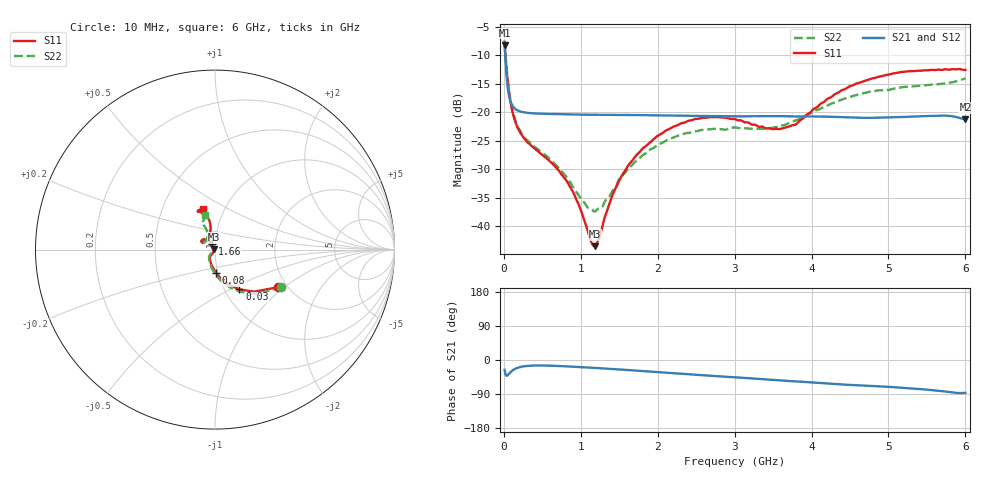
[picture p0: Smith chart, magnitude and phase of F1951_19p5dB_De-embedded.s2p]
! Integrated Device Technology
! Corporate Headquarters
! 6024 Silver Creek Valley Road
! San Jose, CA 95138  USA
! Phone:  1-408-284-8200
! Toll Free:  1-800-223-1366
! Webpage:  http://www.idt.com/
! Timing and RF Division
! 515 Groton Road, Suite 102
! Westford, MA 01886-6024
! Device:  F1951
! Description: 6-bit 0.5 dB Digital Step Attenuator
! Frequency:  100.0 -  4000.00 MHz
! Package:  4x4 mm Thin QFN Plastic Package: 24 pin
! Ports:  2 RF, 6 DC
!  Pin  1  = NC
!  Pin  2  = RF1  =  Port 1
!  Pin  3  = GND
!  Pin  4  = NC
!  Pin  5  = Serial Data Out (SDO)
!  Pin  6  = NC
!  Pin  7  = Reset Bar ( RSTb)
!  Pin  8  = Clock (CLK)
!  Pin  9  = Chip Select Bar (CSb)
!  Pin 10  = NC
!  Pin 11  = Serial Data In (SDI)
!  Pin 12  = NC
!  Pin 13  = NC
!  Pin 14  = VDD
!  Pin 15  = NC
!  Pin 16  = GND
!  Pin 17  = RF2  =  Port 2
!  Pin 18  = NC
!  Pin 19  = GND
!  Pin 20  = GND
!  Pin 21  = GND
!  Pin 22  = GND
!  Pin 23  = GND
!  Pin 24  = GND
! State:  39
! Atten State:  19.5 dB
! Voltage:  +3.30 Volts
! Current:  0.485 mA
! Data:  The device was measured on a F195X evaluation board which has
!  individual transmission lines to the RF pins.  Data was collected
!  de-embedded using a Automatic Fixture Removal [AFR] (Keysight Technologies).
!  The reference plane is the edge of the package pin.
! Misc:  Lot Code  1225BCA
!  Action Tracker AT0399
! Date Measured:  2018-09-13
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# GHz S dB R 50
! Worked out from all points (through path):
!   600 points, 10 MHz to 6 GHz, reference 50 ohm
!   highest |S21| = -8.24 dB at 10 MHz (marker M1); lowest = -21.3 dB at 6 GHz (marker M2)
!   group delay of S21, straight-line fit = 34.4 ps
!   lowest |S11| = -43.5 dB at 1.18 GHz (marker M3), VSWR 1.01, Z = 49.3 + j0.0603 ohm
!   |S11| at or under -10 dB: 20.58 MHz to end of sweep
!   |S22| runs from -37.4 to -7.4 dB; largest |S21 - S12| = 0.00025
!   S11 on the Smith chart (normalised r, x): 10 MHz: 1.79, -0.90; 30 MHz: 1.17, -0.56; 80 MHz: 0.98, -0.26; 1.66 GHz: 0.97, +0.06; 6 GHz: 0.80, +0.38
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0.01  -7.75 -30.8  -8.24 -25.9  -8.25 -25.9  -7.44 -29.6
0.03  -11.71 -58.5  -12.70 -41.1  -12.70 -41.1  -11.28 -59.5
0.08  -17.71 -87.1  -17.82 -33.7  -17.82 -33.7  -17.43 -89.8
0.15  -21.73 -105.3  -19.45 -23.0  -19.45 -23.0  -21.47 -108.4
0.25  -24.34 -117.6  -20.00 -17.0  -20.00 -17.0  -24.10 -122.0
0.72  -30.34 -123.7  -20.36 -15.8  -20.35 -15.9  -29.88 -136.4
0.88  -33.51 -124.3  -20.40 -17.5  -20.40 -17.5  -32.67 -141.1
1.01  -37.56 -130.0  -20.44 -18.9  -20.44 -18.9  -35.35 -150.1
1.13  -42.52 -158.5  -20.45 -20.2  -20.45 -20.2  -36.91 -168.8
1.18  -43.49 174.8  -20.46 -20.8  -20.46 -20.8  -37.42 -180.0
1.24  -42.01 145.3  -20.45 -21.5  -20.46 -21.5  -36.89 168.1
1.43  -33.94 116.8  -20.49 -24.1  -20.48 -24.1  -33.52 140.4
1.66  -28.68 116.8  -20.51 -27.1  -20.51 -27.2  -29.40 130.9
2.01  -24.07 125.7  -20.57 -32.1  -20.57 -32.1  -25.65 133.5
2.49  -21.18 139.7  -20.66 -38.8  -20.65 -38.8  -23.33 141.3
3.01  -21.24 150.4  -20.73 -45.9  -20.74 -45.8  -22.68 145.1
3.58  -22.97 130.1  -20.71 -53.5  -20.71 -53.6  -22.45 127.5
3.79  -22.19 114.1  -20.76 -56.5  -20.76 -56.4  -21.46 120.6
4.01  -19.68 104.4  -20.76 -59.4  -20.76 -59.4  -20.08 115.2
4.49  -15.52 101.2  -20.92 -65.6  -20.92 -65.6  -17.38 113.7
5.01  -13.41 109.4  -20.93 -71.0  -20.93 -70.9  -16.10 116.5
6  -12.61 106.5  -21.26 -86.6  -21.26 -86.6  -14.09 105.7
